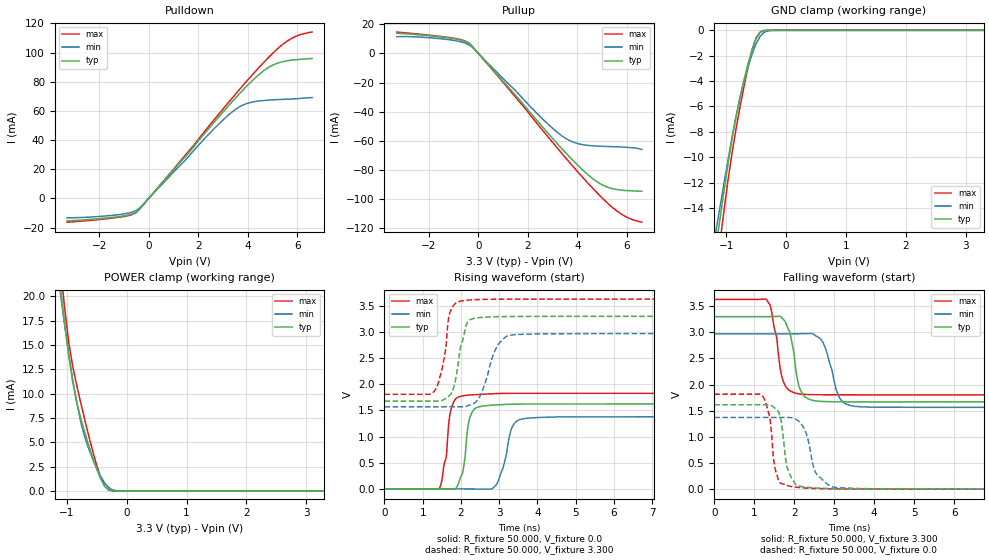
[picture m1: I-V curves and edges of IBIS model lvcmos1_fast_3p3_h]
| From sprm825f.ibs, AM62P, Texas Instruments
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|   fast_3p3_h
[Model]   lvcmos1_fast_3p3_h
Model_type I/O
Polarity   Non-Inverting
Enable   Active-High
Vinl = 0
Vinh = 0.8
Vmeas = 1.65
Vref = 3.3
Cref = 2pF
Rref = 100000
|   typ   min   max
C_comp   3.477pF   3.396pF   3.491pF
[Voltage Range]   3.3   2.97   3.63
[Temperature Range]   27   150   -40
[Pullup Reference]   3.3   2.97   3.63
[Pulldown Reference]   0   0   0
[Power Clamp Reference]   3.3   2.97   3.63
[GND Clamp Reference]   0   0   0
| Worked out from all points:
|   slope of the pulldown table from 0 to 0.495 V, typ, clamps not added: 51.6 ohm
|   slope of the pullup table from 0 to 0.495 V, typ, clamps not added: 52.3 ohm
|   GND clamp passes 1 mA (typ) near -0.53 V on its own axis
|   POWER clamp passes 1 mA (typ) near -0.41 V on its own axis
|   rising waveform, R_fixture 50.000, V_fixture 0.0: 20-80 % time 158ps typ, 269ps min, 184ps max; typ from 0 V to 1.62 V
|   rising waveform, R_fixture 50.000, V_fixture 3.300: 20-80 % time 255ps typ, 375ps min, 216ps max; typ from 1.68 V to 3.3 V
|   falling waveform, R_fixture 50.000, V_fixture 3.300: 20-80 % time 211ps typ, 294ps min, 223ps max; typ from 3.3 V to 1.67 V
|   falling waveform, R_fixture 50.000, V_fixture 0.0: 20-80 % time 189ps typ, 291ps min, 171ps max; typ from 1.61 V to 0 V
[Pulldown]
|Voltage   I(typ)   I(min)   I(max)
-3.3V     -15.39mA   -13.32mA   -16.31mA
-1.2V     -12.47mA   -11.1mA    -12.94mA
-500mV    -9.172mA   -8.138mA   -9.6mA
1.6V      30.91mA    28.58mA    32.15mA
2.7V      53.34mA    48.8mA     55.15mA
3.6V      70.58mA    62.12mA    73.39mA
4V        77.71mA    65.27mA    81.22mA
4.4V      84.18mA    66.7mA     88.81mA
5V        91.35mA    67.61mA    99.41mA
5.4V      93.72mA    67.94mA    105.5mA
5.8V      94.91mA    68.22mA    110mA
6.6V      95.98mA    69.15mA    114.1mA
[Pullup]
|Voltage   I(typ)   I(min)   I(max)
-3.3V     13.92mA    11.59mA    14.75mA
-1.4V     11.14mA    9.957mA    11.49mA
-800mV    9.572mA    8.415mA    9.866mA
-400mV    7.09mA     6.102mA    7.413mA
900mV     -17.21mA   -15.55mA   -17.88mA
2.6V      -50.75mA   -45.22mA   -53.02mA
3.5V      -67.96mA   -58.18mA   -71.41mA
4.1V      -78.42mA   -62.41mA   -83.18mA
4.6V      -85.96mA   -63.54mA   -92.45mA
5V        -90.46mA   -63.93mA   -99.52mA
5.8V      -94.17mA   -64.43mA   -110.9mA
6.6V      -94.93mA   -66.09mA   -116.2mA
[GND_clamp]
|Voltage   I(typ)   I(min)   I(max)
-3.3V     -113.8mA   -82.24mA   -159mA
-1.167V   -17.01mA   -15.72mA   -19.2mA
-1.1V     -14.77mA   -13.85mA   -16.61mA
-1.033V   -12.58mA   -11.98mA   -14.1mA
-900mV    -8.5mA     -8.402mA   -9.615mA
-767mV    -5.246mA   -5.261mA   -6.001mA
-567mV    -1.506mA   -1.867mA   -1.552mA
-500mV    -657.8uA   -1.062mA   -588.9uA
-433mV    -173.4uA   -477.6uA   -123.4uA
-367mV    -24.15uA   -156.5uA   -9.386uA
-233mV    -388.4nA   -8.093uA   -215nA
3.3V      0A         0A         0A
[POWER_clamp]
|Voltage   I(typ)   I(min)   I(max)
-3.3V     168.5mA    143.2mA    197.8mA
-1.1V     20.63mA    20.02mA    22.62mA
-1.033V   17.13mA    16.97mA    18.69mA
-967mV    13.91mA    14.07mA    15.32mA
-900mV    11.2mA     11.41mA    12.78mA
-767mV    7.499mA    7.086mA    9.065mA
-633mV    4.696mA    4.33mA     5.68mA
-500mV    2.241mA    2.328mA    2.652mA
-367mV    494.4uA    819.9uA    490.6uA
-300mV    111.5uA    353.3uA    87.6uA
-100mV    169.5nA    4.694uA    107.5nA
3.3V      0A         0A         0A
[Ramp]
| variable   typ   min   max
dV/dt_r   0.975/0.158n   0.829/0.269n   1.096/0.184n
dV/dt_f   0.978/0.210n   0.843/0.294n   1.095/0.223n
R_load = 50.000
[Rising Waveform]
R_fixture= 50.000
V_fixture= 0.0
V_fixture_min= 0.0
V_fixture_max= 0.0
|time   V(typ)   V(min)   V(max)
0s        1.789uV    19uV       2.438uV
1.433ns   -523.6uV   87.95uV    3.462mV
1.729ns   -3.136mV   35.56uV    1.487V
1.997ns   237.2mV    -208.9uV   1.771V
2.219ns   1.331V     -1.478mV   1.794V
2.469ns   1.57V      -3.455mV   1.806V
2.947ns   1.607V     108.6mV    1.823V
3.335ns   1.619V     1.174V     1.827V
3.585ns   1.622V     1.335V     1.827V
10ns      1.625V     1.381V     1.827V
[Rising Waveform]
R_fixture= 50.000
V_fixture= 3.300
V_fixture_min= 2.970
V_fixture_max= 3.630
|time   V(typ)   V(min)   V(max)
0s        1.678V     1.57V      1.809V
1.296ns   1.678V     1.57V      1.863V
1.506ns   1.69V      1.57V      2.29V
1.679ns   1.773V     1.57V      3.277V
1.773ns   1.863V     1.57V      3.469V
1.983ns   2.692V     1.57V      3.589V
2.22ns    3.228V     1.604V     3.612V
2.94ns    3.292V     2.718V     3.627V
3.26ns    3.296V     2.936V     3.628V
10ns      3.3V       2.97V      3.63V
[Falling Waveform]
R_fixture= 50.000
V_fixture= 3.300
V_fixture_min= 2.970
V_fixture_max= 3.630
|time   V(typ)   V(min)   V(max)
0s        3.3V       2.97V      3.63V
1.31ns    3.3V       2.97V      3.631V
1.433ns   3.302V     2.97V      3.416V
1.776ns   3.206V     2.97V      1.984V
2.061ns   2.186V     2.972V     1.831V
2.244ns   1.786V     2.975V     1.813V
2.71ns    1.678V     2.823V     1.806V
3.111ns   1.672V     1.785V     1.805V
3.371ns   1.671V     1.606V     1.805V
10ns      1.669V     1.565V     1.804V
[Falling Waveform]
R_fixture= 50.000
V_fixture= 0.0
V_fixture_min= 0.0
V_fixture_max= 0.0
|time   V(typ)   V(min)   V(max)
0s        1.614V     1.371V     1.816V
1.211ns   1.614V     1.371V     1.782V
1.389ns   1.612V     1.371V     1.367V
1.499ns   1.562V     1.371V     496.9mV
1.625ns   1.447V     1.371V     140mV
1.863ns   327.4mV    1.371V     61.18mV
2.212ns   45.58mV    1.209V     25.89mV
2.533ns   23.69mV    322.1mV    13.2mV
2.977ns   10.39mV    39.21mV    6.392mV
10ns      58.09uV    126.4uV    35.71uV
